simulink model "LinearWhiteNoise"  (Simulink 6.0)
settings: Solver=ode45  SolverMode=SingleTasking  StartTime=0.0  StopTime=5.0  RelTol=1e-3  AbsTol=1e-6

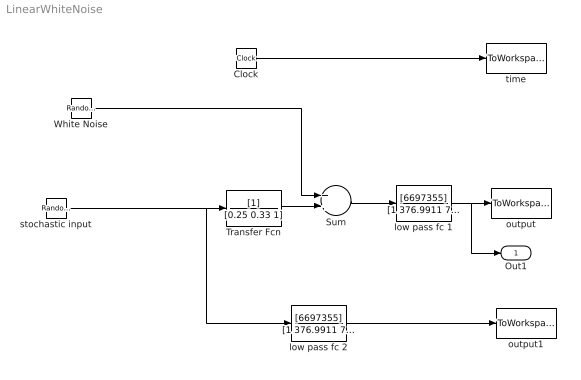
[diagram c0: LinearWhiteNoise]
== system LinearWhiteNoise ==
  Clock : Clock
  Sum : Sum
  Transfer Fcn : TransferFcn  Denominator=[0.25 0.33 1]
  White Noise : RandomNumber  Variance=0.01  Seed=61  SampleTime=0.01
  low pass fc 1 : TransferFcn  Numerator=[6697355]  Denominator=[1 376.9911 71061.15 6697355]
  low pass fc 2 : TransferFcn  Numerator=[6697355]  Denominator=[1 376.9911 71061.15 6697355]
  output : ToWorkspace  VariableName=y  SampleTime=0.01  SaveFormat=Array
  output1 : ToWorkspace  VariableName=u  SampleTime=0.01  SaveFormat=Array
  stochastic input : RandomNumber  Seed=28  SampleTime=0.01
  time : ToWorkspace  VariableName=t  SampleTime=0.01  SaveFormat=Array
  Out1 : Outport
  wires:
  Transfer Fcn/1 -> Sum/2
  Clock/1 -> time/1
  Sum/1 -> low pass fc 1/1
  stochastic input/1 -> Transfer Fcn/1, low pass fc 2/1
  White Noise/1 -> Sum/1
  low pass fc 2/1 -> output1/1
  low pass fc 1/1 -> output/1, Out1/1
